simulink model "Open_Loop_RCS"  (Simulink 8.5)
settings: Solver=ode4  StartTime=0.0  StopTime=3000  FixedStep=Ts  RelTol=1e-3
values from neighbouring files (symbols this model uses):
  Na_max = 0.636/(deadband(1)*d2r)    [start.m]    (also in Dead_Band_DF.m = 72.8802315406; start2.m; start3.m)
  Th = 20    [start.m]    (also in start1.m; start2.m; start3.m)
  wo = 0.0011    [start.m]    (also in start1.m; start2.m; start3.m)
undefined symbols (not defined in the file or in its folder): Af, Bf, Cf, Df, JSel_ln, Mix, UnitV

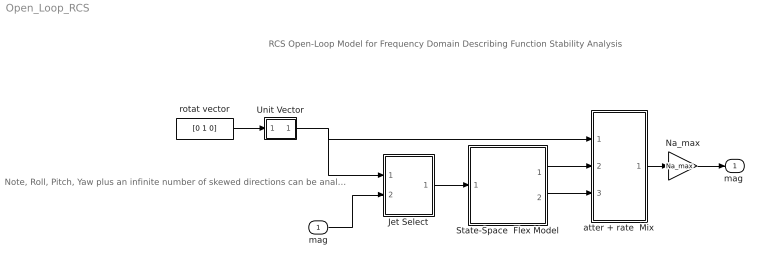
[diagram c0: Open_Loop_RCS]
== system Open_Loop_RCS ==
  note: RCS Open-Loop Model for Frequency Domain Describing Function Stability Analysis
  note: Note, Roll, Pitch, Yaw plus an infinite number of skewed directions can be analyzed for Stability Each direction corresponds to a unique set of thrusters
  mag : Inport  PortDimensions=1
  Jet Select : Subsystem
  Na_max : Gain  Gain=Na_max
  State-Space  Flex Model : Subsystem
  Unit Vector : Subsystem
  atter + rate  Mix : Subsystem
  rotat vector : Constant  Value=[0 1 0]
  "mag " : Outport
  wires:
  State-Space  Flex Model/1(att-lv) -> atter + rate  Mix/2(atter)
  State-Space  Flex Model/2(w-lv) -> atter + rate  Mix/3(rater)
  mag/1 -> Jet Select/2(mag)
  Unit Vector/1(U) -> Jet Select/1(Udir), atter + rate  Mix/1(Udir)
  rotat vector/1 -> Unit Vector/1(V)
  atter + rate  Mix/1(mag) -> Na_max/1
  Na_max/1 -> "mag "/1
  Jet Select/1(th(i)) -> State-Space  Flex Model/1(Th(i))

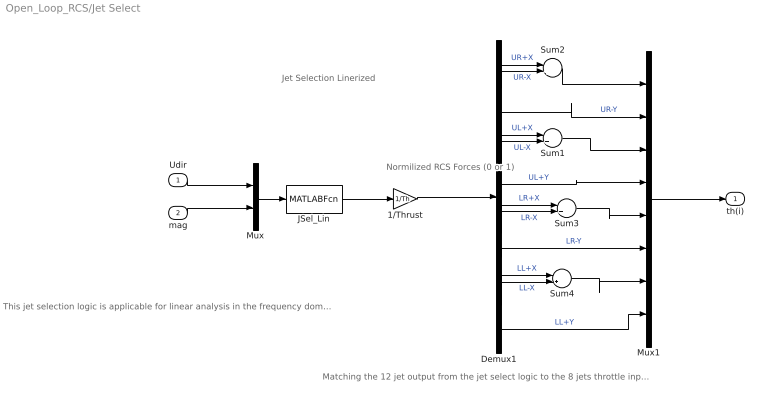
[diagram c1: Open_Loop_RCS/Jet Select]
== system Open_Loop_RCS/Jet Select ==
  note: Jet Selection Linerized
  note: Normilized RCS Forces (0 or 1)
  note: This jet selection logic is applicable for linear analysis in the frequency domain using the Describing Function. Positive and Negative acceleration jets are all used in this linearized version of the jet selection logic. The positive acceleration jets apply positive thrusts, and the negative acceleration jets apply negative thrusts. This creates a more symmetrical system. The jet thrusts are reduced to half since the acceleration is doubled by the negative firing jets
  note: Matching the 12 jet output from the jet select logic to the 8 jets throttle input of the vehicle model
  Udir : Inport
  mag : Inport  Port=2
  1/Thrust : Gain  Gain=1/Th
  Demux1 : Demux  Outputs=nt
  JSel_Lin : MATLABFcn  MATLABFcn=JSel_ln( u(1:3), u(4) )  OutputDimensions=nt
  Mux : Mux  Inputs="[3  1]"
  Mux1 : Mux  Inputs=8
  Sum{1..4} (4 alike) : Sum  Inputs=|+-
  th(i) : Outport
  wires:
  Mux/1 -> JSel_Lin/1
  Udir/1 -> Mux/1
  mag/1 -> Mux/2
  Demux1/1 -> Sum2/1  "UR+X"
  Demux1/2 -> Sum2/2  "UR-X"
  Demux1/4 -> Sum1/1  "UL+X"
  Demux1/5 -> Sum1/2  "UL-X"
  Demux1/7 -> Sum3/1  "LR+X"
  Demux1/8 -> Sum3/2  "LR-X"
  Demux1/10 -> Sum4/1  "LL+X"
  Demux1/11 -> Sum4/2  "LL-X"
  Demux1/3 -> Mux1/2  "UR-Y"
  Sum2/1 -> Mux1/1
  Demux1/6 -> Mux1/4  "UL+Y"
  Demux1/9 -> Mux1/6  "LR-Y"
  Sum4/1 -> Mux1/7
  Demux1/12 -> Mux1/8  "LL+Y"
  1/Thrust/1 -> Demux1/1
  JSel_Lin/1 -> 1/Thrust/1
  Sum3/1 -> Mux1/5
  Sum1/1 -> Mux1/3
  Mux1/1 -> th(i)/1

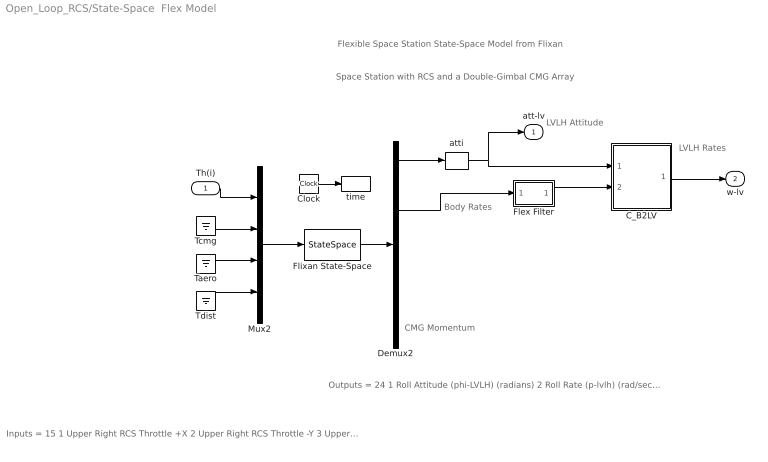
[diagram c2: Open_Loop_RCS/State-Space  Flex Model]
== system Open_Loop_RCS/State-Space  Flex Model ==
  note: Space Station with RCS and a Double-Gimbal CMG Array
  note: Flexible Space Station State-Space Model from Flixan
  note: LVLH Attitude
  note: LVLH Rates
  note: Outputs = 24 1 Roll Attitude (phi-LVLH) (radians) 2 Roll Rate (p-lvlh) (rad/sec) 3 Pitch Attitude (thet-LVLH) (radians) 4 Pitch Rate (q-lvlh) (rad/sec) 5 Yaw Attitude (psi-LVLH) (radians) 6 Yaw Rate (r-lvlh) (rad/sec) 7 Angle of attack, alfa, (radians) 8 Angle of sideslip, beta, (radian) 9 Change in Altitude, delta-h, (feet) 10 Forward Acceleration (V-dot) (ft/sec) 11 Cross Range Velocity (Vcr) (ft/sec) 12 Rate-Gyro # 1, Roll Rate (Body) (rad/sec) 13 Rate-Gyro # 2, Pitch Rate (Body) (rad/sec) 14 Rate-Gyro # 3, Yaw Rate (Body) (rad/sec) 15 Gyro # 4, Roll Attitude (Body) (radians) 16 Gyro # 5, Pitch Attitude (Body) (radians) 17 Gyro # 6, Yaw Attitude (Body) (radians) 18 Accelerom # 1, (along X), (ft/sec^2) Translat. Accelerat. 19 Accelerom # 2, (along Z), (ft/sec^2) Translat. Accelerat. 20 Accelerom # 3, (along X), (ft/sec^2) Translat. Accelerat. 21 Accelerom # 4, (along Z), (ft/sec^2) Translat. Accelerat. 22 Double Gimbal CMG Momentum Change in X-axis (ft-lb-sec) 23 Double Gimbal CMG Momentum Change in Y-axis (ft-lb-sec) 24 Double Gimbal CMG Momentum Change in Z-axis (ft-lb-sec)
  note: Inputs = 15 1 Upper Right RCS Throttle +X 2 Upper Right RCS Throttle -Y 3 Upper Left RCS Throttle +X 4 Upper Left RCS Throttle +Y 5 Lower Right RCS Throttle +X 6 Lower Right RCS Throttle -Y 7 Lower Left RCS Throttle +X 8 Lower Left RCS Throttle +Y 9 Double Gimbal CMG Torque in the X-axis (ft-lb) 10 Double Gimbal CMG Torque in the Y-axis (ft-lb) 11 Double Gimbal CMG Torque in the Z-axis (ft-lb) 12 External Torque Input 1 (ft-lb), direct: 13 External Torque Input 2 (ft-lb), direct: 14 External Torque Input 3 (ft-lb), direct: 15 Ext Torque Direct.=(0.197, -0.5964, -0.7782)
  note: CMG Momentum
  note: Body Rates
  Th(i) : Inport
  C_B2LV : Subsystem
  Clock : Clock
  Demux2 : Demux  Outputs=[11, 3, 3, 4, 3]
  Flex Filter : Subsystem
  Flixan State-Space : StateSpace  A=Af  B=Bf  C=Cf  D=Df  X0=0
  Mux2 : Mux  Inputs=[8, 3, 3, 1]
  Taero : Ground
  Tcmg : Ground
  Tdist : Ground
  atti : Selector  InputPortWidth=11  Indices=[1 3 5]
  time : ToWorkspace  VariableName=time  SampleTime=-1
  att-lv : Outport
  w-lv : Outport  Port=2
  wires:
  Demux2/2 -> Flex Filter/1(I)
  Demux2/1 -> atti/1
  Th(i)/1 -> Mux2/1
  Clock/1 -> time/1
  Tcmg/1 -> Mux2/2
  Flixan State-Space/1 -> Demux2/1
  Mux2/1 -> Flixan State-Space/1
  Taero/1 -> Mux2/3
  Tdist/1 -> Mux2/4
  atti/1 -> att-lv/1, C_B2LV/1(atti)
  Flex Filter/1(O) -> C_B2LV/2(wb)
  C_B2LV/1(wlv) -> w-lv/1

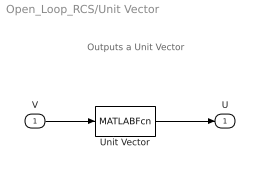
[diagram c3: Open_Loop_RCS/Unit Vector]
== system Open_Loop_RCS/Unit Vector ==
  note: Outputs a Unit Vector
  V : Inport
  Unit Vector : MATLABFcn  MATLABFcn=UnitV( u(1:3) )  OutputDimensions=3
  U : Outport
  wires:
  Unit Vector/1 -> U/1
  V/1 -> Unit Vector/1

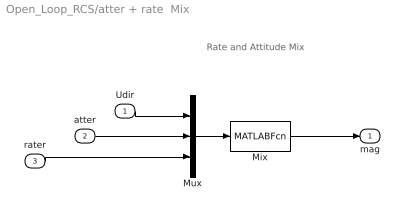
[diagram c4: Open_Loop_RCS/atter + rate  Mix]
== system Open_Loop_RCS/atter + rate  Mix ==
  note: Rate and Attitude Mix
  Udir : Inport
  atter : Inport  Port=2
  rater : Inport  Port=3
  Mix : MATLABFcn  MATLABFcn=Mix( u(1:3), u(4:6), u(7:9) )  OutputDimensions=1
  Mux : Mux  Inputs="[3  3  3]"
  mag : Outport
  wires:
  rater/1 -> Mux/3
  Mux/1 -> Mix/1
  Udir/1 -> Mux/1
  atter/1 -> Mux/2
  Mix/1 -> mag/1

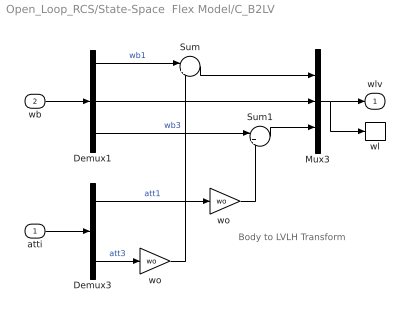
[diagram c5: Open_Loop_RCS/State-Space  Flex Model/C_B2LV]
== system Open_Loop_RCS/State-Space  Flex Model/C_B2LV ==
  note: Body to LVLH Transform
  atti : Inport  PortDimensions=3
  wb : Inport  Port=2  PortDimensions=3
  Demux1 : Demux  Outputs=3
  Demux3 : Demux  Outputs=3
  Mux3 : Mux  Inputs=3
  Sum : Sum  Inputs=|++
  Sum1 : Sum  Inputs=|+-
  wl : ToWorkspace  VariableName=wl  SampleTime=-1
  wo : Gain  Gain=wo
  "wo " : Gain  Gain=wo
  wlv : Outport
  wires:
  Demux1/1 -> Sum/1  "wb1"
  Sum/1 -> Mux3/1
  Demux3/3 -> wo/1  "att3"
  Sum1/1 -> Mux3/3
  atti/1 -> Demux3/1
  wb/1 -> Demux1/1
  Mux3/1 -> wlv/1, wl/1
  Demux3/1 -> "wo "/1  "att1"
  Demux1/2 -> Mux3/2
  wo/1 -> Sum/2
  Demux1/3 -> Sum1/1  "wb3"
  "wo "/1 -> Sum1/2

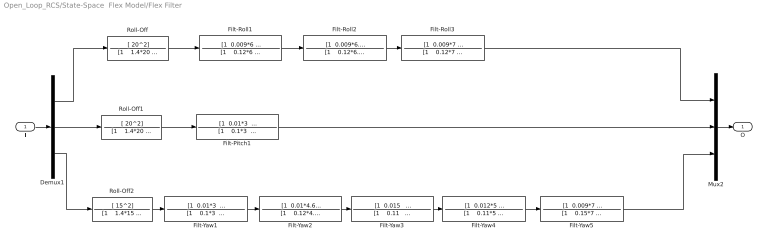
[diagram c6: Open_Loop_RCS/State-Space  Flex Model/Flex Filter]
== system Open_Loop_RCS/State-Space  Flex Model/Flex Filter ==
  I : Inport
  Demux1 : Demux  Outputs=3
  Filt-Pitch1 : TransferFcn  Numerator="[1  0.01*3   3.07^2]"  Denominator="[1    0.1*3    3.07^2]"
  Filt-Roll1 : TransferFcn  Numerator="[1  0.009*6   5.85^2]"  Denominator="[1    0.12*6    5.85^2]"
  Filt-Roll2 : TransferFcn  Numerator="[1  0.009*6.4   6.46^2]"  Denominator="[1    0.12*6.4    6.46^2]"
  Filt-Roll3 : TransferFcn  Numerator="[1  0.009*7   7.51^2]"  Denominator="[1    0.12*7    7.51^2]"
  Filt-Yaw1 : TransferFcn  Numerator="[1  0.01*3   3.07^2]"  Denominator="[1    0.1*3    3.07^2]"
  Filt-Yaw2 : TransferFcn  Numerator="[1  0.01*4.6   4.6^2]"  Denominator="[1    0.12*4.6    4.6^2]"
  Filt-Yaw3 : TransferFcn  Numerator="[1  0.015   1.14^2]"  Denominator="[1    0.11    1.14^2]"
  Filt-Yaw4 : TransferFcn  Numerator="[1  0.012*5   5.21^2]"  Denominator="[1    0.11*5    5.21^2]"
  Filt-Yaw5 : TransferFcn  Numerator="[1  0.009*7   6.83^2]"  Denominator="[1    0.15*7    6.83^2]"
  Mux2 : Mux  Inputs=3
  Roll-Off : TransferFcn  Numerator=[ 20^2]  Denominator="[1    1.4*20    20^2]"
  Roll-Off1 : TransferFcn  Numerator=[ 20^2]  Denominator="[1    1.4*20    20^2]"
  Roll-Off2 : TransferFcn  Numerator=[ 15^2]  Denominator="[1    1.4*15    15^2]"
  O : Outport
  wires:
  I/1 -> Demux1/1
  Mux2/1 -> O/1
  Demux1/1 -> Roll-Off/1
  Demux1/3 -> Roll-Off2/1
  Demux1/2 -> Roll-Off1/1
  Roll-Off/1 -> Filt-Roll1/1
  Roll-Off2/1 -> Filt-Yaw1/1
  Roll-Off1/1 -> Filt-Pitch1/1
  Filt-Roll1/1 -> Filt-Roll2/1
  Filt-Roll2/1 -> Filt-Roll3/1
  Filt-Roll3/1 -> Mux2/1
  Filt-Pitch1/1 -> Mux2/2
  Filt-Yaw1/1 -> Filt-Yaw2/1
  Filt-Yaw2/1 -> Filt-Yaw3/1
  Filt-Yaw3/1 -> Filt-Yaw4/1
  Filt-Yaw4/1 -> Filt-Yaw5/1
  Filt-Yaw5/1 -> Mux2/3
